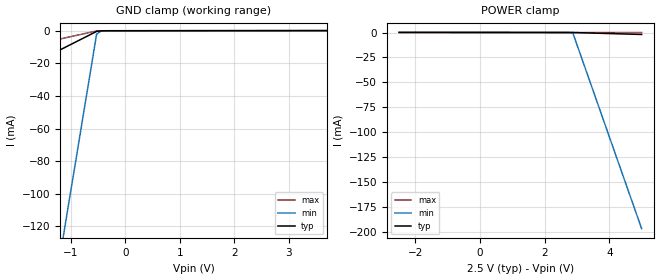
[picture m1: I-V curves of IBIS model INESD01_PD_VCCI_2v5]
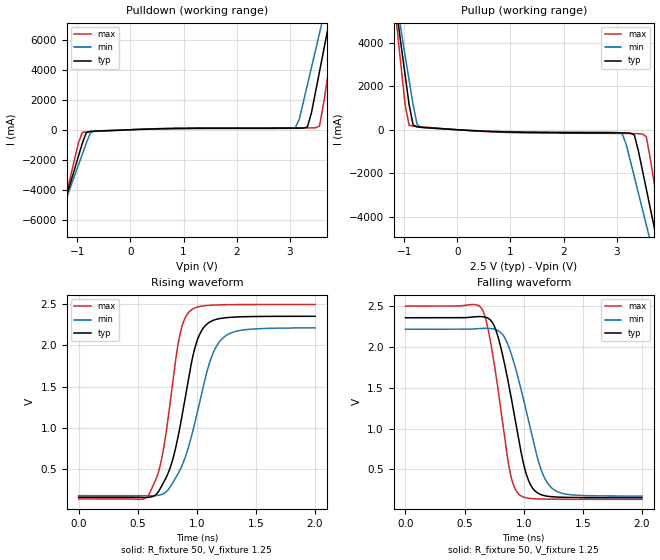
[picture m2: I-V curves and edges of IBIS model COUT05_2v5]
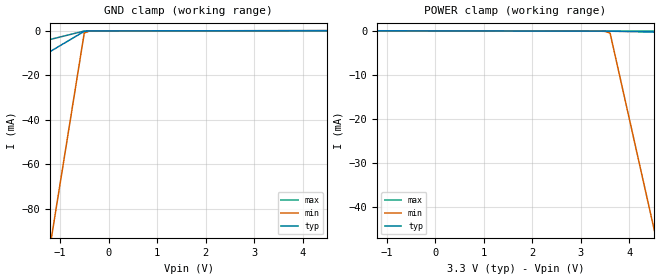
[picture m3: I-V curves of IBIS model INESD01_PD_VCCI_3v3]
|   This file is an IBIS representation of the   |
|   Integrated Device Technology, Inc.   |
|   ICS8304-01   |
|   LOW SKEW, 1-TO-4 LVCMOS/LVTTL INVERTING FANOUT BUFFER   |
[IBIS Ver]   4.1
[File name]   8304_01.ibs
[File Rev]   3.0
[Date]   29 Apr 2009 | Last modified
|   Jul  1 2003   | Generated
[Source]   Originated at Integrated Devices Technology, Inc.
[Disclaimer]
IDT hereby grants the user of this IBIS model a non-exclusive,
nontransferable license to use this IBIS model under the following terms.
Before using this IBIS model, the user should read this license.
If the user does not accept these terms,  the IBIS model should be
returned to IDT within 30 days.
   The user is granted this license only to use the IBIS model and
is not granted rights to sell, load, rent, lease or license the IBIS
model in whole or in part, or in modified form to anyone other than
user. User may modify the IBIS model to suit its specific
applications but rights to derivative works and such modifications
shall belong to IDT.
   This IBIS model is provided on an "AS IS" basis and IDT makes
absolutely no warranty with respect to the information contained
herein. IDT DISCLAIMS AND CUSTOMER WAIVES ALL WARRANTIES, EXPRESS
OR IMPLIED, INCLUDING WARRANTIES OF MERCHANTABILITY OR FITNESS FOR
A PARTICULAR PURPOSE. The entire risk as to quality and performance
is with the Customer. ACCORDINGLY, IN NO EVENT SHALL THE COMPANY BE
LIABLE FOR ANY DAMAGES, WHETHER IN CONTRACT OR TORT,INCLUDING ANY
LOST PROFITS OR OTHER INCIDENTAL, CONSEQUENTIAL, EXEMPLARY, OR
PUNITIVE DAMAGES ARISING OUT OF THE USE OR APPLICATION OF THE IBIS
model provided in this package. Further, IDT reserves the right to
make changes without notice to any product herein to improve
reliability, function, or design. IDT does not convey any license
under patent rights or any other intellectual property rights,
including those of third parties.
   IDT is not obligated to provide maintenance or support
for the licensed IBIS model.
[Copyright]   Copyright 2008 by Integrated Device Technology, Inc.
[Component]   ICS8304AM-01
[Manufacturer] Integrated Devices Technology, Inc.
[Package]
|SOIC 8 Lead
|   typ   min   max
R_pkg   57.05m   55.5m   58.6m
L_pkg   1.769nH   1.570nH   1.968nH
C_pkg   0.269pF   0.252pF   0.286pF
[Pin] signal_name  model_name   R_pin   L_pin   C_pin
1   VDDO   POWER   58.6m   1.968n   0.286p
2   VDD   POWER   55.5m   1.570n   0.252p
3   CLK   INESD01_PD_VCCI   55.5m   1.570n   0.252p
4   GND   GND   56.6m   1.968n   0.286p
5   nQ0   COUT05   58.6m   1.968n   0.286p
6   nQ1   COUT05   55.5m   1.570n   0.252p
7   nQ2   COUT05   55.5m   1.570n   0.252p
8   nQ3   COUT05   56.6m   1.968n   0.286p
[Model Selector] INESD01_PD_VCCI
INESD01_PD_VCCI_2v5  Buffer selection for 2v5
INESD01_PD_VCCI_3v3  Buffer selection for 3v3
[Model Selector] COUT05
COUT05_2v5  Buffer selection for 2v5
COUT05_3v3  Buffer selection for 3v3
| Models and submodels in the file (4): INESD01_PD_VCCI_2v5 (Input), COUT05_2v5 (Output), INESD01_PD_VCCI_3v3 (Input), COUT05_3v3 (Output)
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[Model] INESD01_PD_VCCI_2v5
Model_type   Input
Polarity   Non-Inverting
Vinl = 1.3V
Vinh = 2.0V
|   typ   min   max
C_comp   2pF   1.5pF   2.5pF
|   typ   min   max
[Voltage range]  2.5V   2.375V   2.625V
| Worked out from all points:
|   GND clamp passes 1 mA (typ) near -0.56 V on its own axis
[GND_clamp]
|Voltage I(typ)   I(min)   I(max)
-2.5V     -33.66mA   -401.1mA   -14.61mA
-1.136V   -10.64mA   -124.9mA   -4.585mA
-1.061V   -9.365mA   -109.5mA   -4.028mA
-530.3mV  -415.4uA   -2.119mA   -130uA
-454.5mV  -90.52uA   -342uA     -24.79uA
5V        97.98uA    94.31uA    101.7uA
[POWER_clamp]
|Voltage   I(typ)   I(min)   I(max)
-2.5V     97.98uA    91.95uA    104.2uA
2.652V    -2.989uA   -11.36uA   -539.2nA
2.879V    -21.06uA   -1.086mA   -5.176uA
5V        -1.966mA   -196.9mA   -55.09uA
[Model] COUT05_2v5
Model_type   Output
Polarity   Non-Inverting
|   typ   min   max
C_comp   2pF   1.5pF   2.5pF
Vmeas = 1.25V
Rref = 50
Cref = 50
Vref = 1.25V
|   typ   min   max
[Voltage range]   2.5V   2.375V   2.625V
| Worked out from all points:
|   slope of the pulldown table from 0 to 0.375 V, typ, clamps not added: 7.84 ohm
|   slope of the pullup table from 0 to 0.375 V, typ, clamps not added: 7.17 ohm
|   rising waveform, R_fixture 50, V_fixture 1.25: 20-80 % time 181ps typ, 224ps min, 142ps max; typ from 0.154 V to 2.35 V
|   falling waveform, R_fixture 50, V_fixture 1.25: 20-80 % time 175ps typ, 211ps min, 143ps max; typ from 2.35 V to 0.154 V
[Pulldown]
|Voltage   I (typ)   I (min)   I (max)
-2.5V     -19.75A    -17.35A    -23.82A
-1.439V   -7.206A    -6.887A    -7.808A
-1.364V   -6.308A    -6.139A    -6.662A
-909.1mV  -921.7mA   -1.65A     -183.6mA
-833.3mV  -199.2mA   -901.6mA   -138mA
-681.8mV  -95.6mA    -94.51mA   -111.1mA
3.106V    103.9mA    147.7mA    121.5mA
3.333V    187.7mA    3.001A     122.2mA
3.561V    3.866A     6.429A     248.4mA
3.712V    6.611A     8.717A     3.472A
3.864V    9.357A     11A        6.981A
5V        29.99A     28.19A     33.35A
[Pullup]
|Voltage   I (typ)   I (min)   I (max)
-2.5V     30.11A     26.42A     36.38A
-1.136V   5.3A       5.738A     4.69A
-1.061V   3.921A     4.589A     2.928A
-909.1mV  1.162A     2.291A     208.3mA
-681.8mV  112.8mA    108.8mA    133.2mA
3.106V    -144.5mA   -188.3mA   -168.5mA
3.333V    -240.4mA   -2.164A    -175.3mA
3.485V    -1.852A    -3.654A    -191.8mA
3.561V    -2.745A    -4.399A    -320.2mA
3.712V    -4.534A    -5.89A     -2.513A
3.864V    -6.324A    -7.381A    -4.797A
5V        -19.75A    -18.57A    -21.94A
[Ramp]
|   typ   min   max
dV/dt_r   1.763/0.291n   1.634/0.358n   1.895/0.227n
dV/dt_f   1.772/0.26n   1.642/0.314n   1.906/0.211n
R_load =   50.0000
[Rising Waveform]
R_fixture = 50
V_fixture = 1.25   |Vcc_typ
V_fixture_min = 1.1875 |Vcc_min
V_fixture_max = 1.3125 |Vcc_max
C_fixture = 0.0p
| Time   typ   min   max
0s        154.1mV    173.3mV    133.8mV
594.6ps   153.1mV    171mV      187.8mV
694.7ps   270mV      184.1mV    568.7mV
782.8ps   548.4mV    298.9mV    1.397V
860.9ps   1.034V     493.9mV    2.157V
948.9ps   1.748V     863.7mV    2.427V
1.049ns   2.2V       1.466V     2.48V
1.131ns   2.301V     1.885V     2.49V
1.223ns   2.334V     2.094V     2.495V
2ns       2.355V     2.214V     2.498V
[Falling Waveform]
R_fixture = 50
V_fixture = 1.25   |Vcc_typ
V_fixture_min = 1.1875 |Vcc_min
V_fixture_max = 1.3125 |Vcc_max
C_fixture = 0.0p
| Time   typ   min   max
0s        2.355V     2.214V     2.498V
646.6ps   2.368V     2.225V     2.462V
702.7ps   2.345V     2.225V     2.186V
780.8ps   2.131V     2.199V     1.501V
882.9ps   1.467V     1.963V     477.1mV
965ps     809.8mV    1.551V     188.8mV
1.065ns   293.1mV    943.2mV    143.1mV
1.149ns   189.4mV    489.6mV    137.3mV
1.235ns   165.9mV    275.2mV    135.3mV
2ns       154.1mV    173.6mV    133.8mV
[Model] INESD01_PD_VCCI_3v3
Model_type   Input
Polarity   Non-Inverting
Vinl = 1.3V
Vinh = 2.0V
|   typ   min   max
C_comp   2pF   1.5pF   2.5pF
|   typ   min   max
[Voltage range]  3.3V   3.15V   3.45V
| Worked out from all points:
|   GND clamp passes 1 mA (typ) near -0.56 V on its own axis
[GND_clamp]
|Voltage I(typ)   I(min)   I(max)
-3.3V     -36.4mA    -382.1mA   -15.22mA
-1.2V     -9.271mA   -96.28mA   -3.853mA
-1.1V     -7.979mA   -82.66mA   -3.312mA
-500mV    -227.8uA   -989.9uA   -65.11uA
-400mV    -30.81uA   -105.6uA   -11.01uA
-300mV    -7.585uA   -16.23uA   -6.189uA
6.6V      129.3uA    124.7uA    134.2uA
[POWER_clamp]
|Voltage   I(typ)   I(min)   I(max)
-3.3V     129.3uA    121.5uA    137.6uA
3.4V      -1.963uA   -9.687uA   1.322uA
3.5V      -4.012uA   -52.24uA   -711.7nA
3.6V      -7.585uA   -433.5uA   -2.745uA
4.5V      -216.6uA   -44.85mA   -21.11uA
4.6V      -239.9uA   -49.78mA   -23.15uA
6.6V      -704.4uA   -148.5mA   -63.97uA
